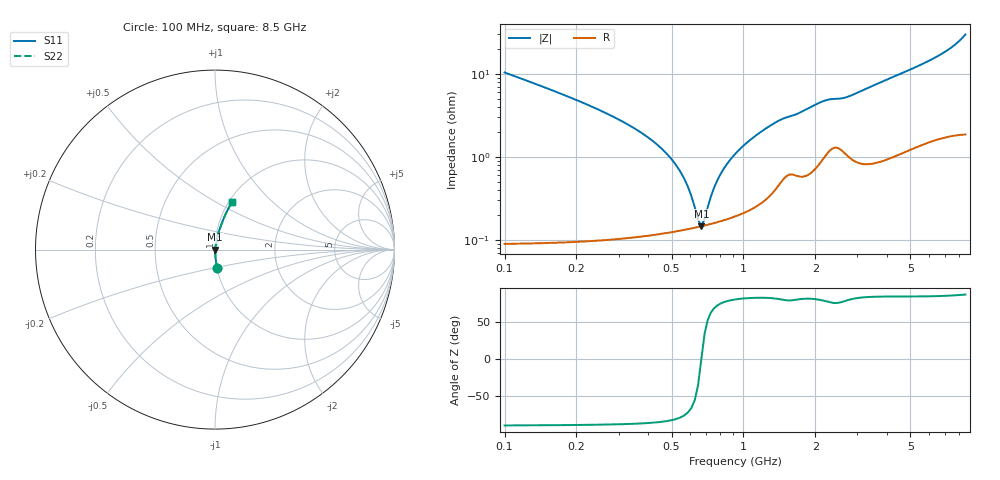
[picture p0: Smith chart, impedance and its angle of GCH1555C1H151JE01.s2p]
!Murata Part Number: GCH1555C1H151JE01
!These Parameters are Measured in Series Mode Connection
!Data Generated on Mar 13, 2026
!  o--ll--o
!Port1  Port2
!  o------o
!Operation Temp=25[degC], DC Bias Voltage=0[V]
!Freq. Start=100[MHz] Stop=9[GHz] 401[Steps]
# Hz S RI R 50
!Freq.(Hz) S11(Real) S11(Imag) S21(Real) S21(Imag) S12(Real) S12(Imag) S22(Real) S22(Imag)
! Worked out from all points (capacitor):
!   401 points, 100 MHz to 8.5 GHz, reference 50 ohm
!   read as one part in series: C = 150 pF near 142 MHz
!   lowest |Z| = 145 mohm at 667 MHz (marker M1)
!   series resonance near 666.7 MHz, so ESL is about 380 pH
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1e8  0.0115 -0.1024  0.9885 0.1024  0.9885 0.1024  0.0115 -0.1024
2.26e8  0.00267 -0.0414  0.9973 0.0414  0.9973 0.0414  0.00267 -0.0414
4.78e8  0.00132 -0.0107  0.9987 0.0107  0.9987 0.0107  0.00132 -0.0107
5.62e8  0.00134 -0.00545  0.9987 0.00545  0.9987 0.00545  0.00134 -0.00545
6.25e8  0.0014 -0.00205  0.9986 0.00205  0.9986 0.00205  0.0014 -0.00205
6.46e8  0.00142 -0.001  0.9986 0.001  0.9986 0.001  0.00142 -0.001
6.67e8  0.00145 1.45e-05  0.9985 -1.45e-05  0.9985 -1.45e-05  0.00145 1.45e-05
6.88e8  0.00148 0.001  0.9985 -0.001  0.9985 -0.001  0.00148 0.001
7.09e8  0.00152 0.00196  0.9985 -0.00196  0.9985 -0.00196  0.00152 0.00196
7.72e8  0.00164 0.00469  0.9984 -0.00469  0.9984 -0.00469  0.00164 0.00469
8.14e8  0.00173 0.00641  0.9983 -0.00641  0.9983 -0.00641  0.00173 0.00641
8.77e8  0.00189 0.00887  0.9981 -0.00887  0.9981 -0.00887  0.00189 0.00887
9.4e8  0.00207 0.0112  0.9979 -0.0112  0.9979 -0.0112  0.00207 0.0112
1.045e9  0.00243 0.015  0.9976 -0.015  0.9976 -0.015  0.00243 0.015
1.192e9  0.00316 0.0199  0.9968 -0.0199  0.9968 -0.0199  0.00316 0.0199
1.507e9  0.00657 0.0288  0.9934 -0.0288  0.9934 -0.0288  0.00657 0.0288
2.179e9  0.0118 0.0452  0.9882 -0.0452  0.9882 -0.0452  0.0118 0.0452
2.914e9  0.0119 0.0551  0.9881 -0.0551  0.9881 -0.0551  0.0119 0.0551
4.3e9  0.0183 0.0903  0.9817 -0.0903  0.9817 -0.0903  0.0183 0.0903
5.707e9  0.0308 0.1276  0.9692 -0.1276  0.9692 -0.1276  0.0308 0.1276
7.114e9  0.0501 0.1773  0.9499 -0.1773  0.9499 -0.1773  0.0501 0.1773
8.5e9  0.0954 0.2643  0.9046 -0.2643  0.9046 -0.2643  0.0954 0.2643
